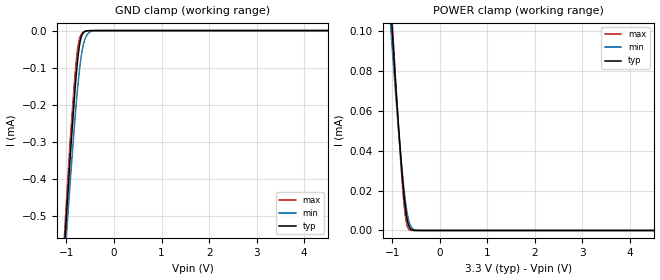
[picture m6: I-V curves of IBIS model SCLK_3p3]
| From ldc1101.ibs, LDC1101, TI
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|   Model
[Model]   SCLK_3p3
Model_type   Input
Vinl = 0.99
Vinh = 2.31
|   typ   min   max
C_comp   0.346pF   0.312pF   0.398pF
[Voltage Range]   3.3   3.14   3.46
[Temperature Range]   27   125   -40
[Power Clamp Reference]   3.3   3.14   3.46
[GND Clamp Reference]   0   0   0
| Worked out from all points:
|   GND clamp passes 1 mA (typ) near -1.23 V on its own axis
[GND Clamp]
|   Voltage   I(typ)   I(min)   I(max)
-3.3V     -5.702mA   -5.303mA   -6.131mA
-1.033V   -570.2uA   -617.1uA   -535.8uA
-1.013V   -529.1uA   -579.7uA   -492uA
-1.003V   -508.7uA   -561.1uA   -470.4uA
-904.2mV  -311.3uA   -380.3uA   -266.6uA
-795.3mV  -122.3uA   -200.4uA   -84.52uA
-755.7mV  -69.89uA   -144.3uA   -40.88uA
-716.1mV  -32.94uA   -96.58uA   -17.99uA
-617.1mV  -3.045uA   -26.08uA   -2.186uA
-528mV    -289.7nA   -5.806uA   -145.9nA
-399.3mV  -15.93nA   -325.5nA   0A
6.6V      0A         0A         0A
[POWER Clamp]
|   Voltage   I(typ)   I(min)   I(max)
-3.3V     1.045mA    925.2uA    1.142mA
-1.082V   131uA      118uA      138.6uA
-933.9mV  75.63uA    70.09uA    77.05uA
-864.6mV  51.47uA    49.4uA     50.07uA
-815.1mV  35.49uA    35.76uA    32.27uA
-775.5mV  23.96uA    25.87uA    19.64uA
-735.9mV  14.17uA    17.25uA    9.527uA
-686.4mV  5.574uA    8.898uA    2.355uA
-627mV    1.157uA    3.071uA    240.8nA
-557.7mV  129.6nA    664nA      9.046nA
-399.3mV  283.4pA    6.598nA    0A
6.6V      0A         0A         0A
